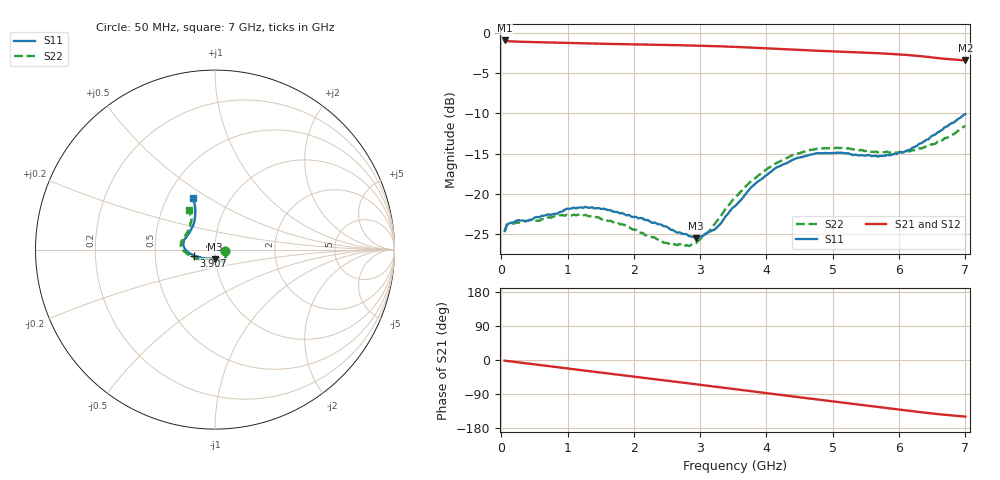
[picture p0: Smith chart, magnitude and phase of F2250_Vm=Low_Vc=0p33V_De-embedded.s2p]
! Integrated Device Technology
! Corporate Headquarters
! 6024 Silver Creek Valley Road
! San Jose, CA 95138  USA
! Phone:  1-408-284-8200
! Toll Free:  1-800-223-1366
! Webpage:  http://www.idt.com/
! Timing and RF Division
! 515 Groton Road, Suite 102
! Westford, MA 01886-6024
! Device:  F2250
! Description: Voltage Variable RF Attenuator
! Frequency:  50.0 -  6000.00 MHz
! Package:  3x3 mm Thin QFN Plastic Package: 16 pin
! Ports:  2 RF, 3 DC
!  Pin  1  = GND
!  Pin  2  = NC
!  Pin  3  = RF1  = Port 1
!  Pin  4  = NC
!  Pin  5  = GND
!  Pin  6  = GND
!  Pin  7  = GND
!  Pin  8  = GND
!  Pin  9  = NC
!  Pin 10  = RF2  = Port 2
!  Pin 11  = NC
!  Pin 12  = GND
!  Pin 13  = GND
!  Pin 14  = VCNTRL
!  Pin 15  = VDD
!  Pin 16  = VMODE
! Vcntrl:  0.330 Volts
! Vmode:  +0.000 Volts
! Vdd:  +3.30  Volts
! Current:  1.119 mA
! Data:  The device was measured on a the F2250 evaluation board which has
!  individual transmission lines to the RF pins.  Data was collected
!  using a calibrated network analyzer.  The evaluation board was
!  de-embedded using a TRL calibration technique.
!  The reference plane is the edge of the package pin.
! Misc:  SN 10
!  Action Tracker AT0258
! Date Measured:  2014-11-26
! Date:  2015-10-15  MJV
! Note:
!  Integrated Device Technology supplies this data as a sample of measured
!  data at the package pin for this product.  Your particular data for this
!  product may vary.
!  Data was taken at 25 degrees C.
!  Integrated Device Technology reserves the right to change this data at anytime.
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# GHz S dB R 50
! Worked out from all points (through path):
!   201 points, 50 MHz to 7 GHz, reference 50 ohm
!   highest |S21| = -0.96 dB at 50 MHz (marker M1); lowest = -3.4 dB at 7 GHz (marker M2)
!   group delay of S21, straight-line fit = 60 ps
!   lowest |S11| = -25.5 dB at 2.934 GHz (marker M3), VSWR 1.11, Z = 49.8 - j5.29 ohm
!   |S11| at or under -10 dB: start of sweep to end of sweep
!   |S22| runs from -26.5 to -11.5 dB; largest |S21 - S12| = 0.00032
!   S11 on the Smith chart (normalised r, x): 50 MHz: 1.12, -0.02; 3.907 GHz: 0.79, -0.05; 7 GHz: 0.67, +0.43
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0.05  -24.58 -9.2  -0.96 -1.8  -0.96 -1.8  -24.72 -9.7
0.08475  -23.77 -9.1  -1.03 -2.5  -1.03 -2.5  -23.84 -9.0
0.15425  -23.54 -11.3  -1.08 -4.0  -1.08 -4.0  -23.61 -10.8
0.57125  -22.88 -28.9  -1.18 -13.1  -1.18 -13.1  -23.34 -29.8
0.884  -22.23 -44.3  -1.24 -19.9  -1.24 -19.9  -22.63 -46.0
1.2315  -21.70 -54.4  -1.32 -27.4  -1.32 -27.4  -22.64 -58.8
1.75275  -22.24 -61.1  -1.41 -38.4  -1.41 -38.4  -23.47 -66.1
2.37825  -23.76 -62.1  -1.50 -51.8  -1.50 -51.8  -25.70 -68.5
2.552  -24.41 -66.1  -1.53 -55.6  -1.53 -55.6  -26.33 -74.2
2.83  -25.22 -80.7  -1.58 -61.7  -1.58 -61.7  -26.45 -92.9
2.93425  -25.51 -89.4  -1.60 -64.0  -1.60 -64.0  -26.11 -101.4
3.21225  -24.44 -118.6  -1.66 -70.2  -1.66 -70.2  -23.77 -126.7
3.525  -21.50 -145.8  -1.76 -77.1  -1.76 -77.1  -20.48 -145.7
3.76825  -19.17 -159.5  -1.85 -82.5  -1.85 -82.5  -18.39 -156.2
3.90725  -18.26 -164.0  -1.90 -85.5  -1.90 -85.5  -17.52 -162.3
4.1505  -16.70 -172.4  -2.00 -90.8  -2.00 -90.8  -16.16 -171.0
4.7065  -15.05 173.2  -2.21 -102.9  -2.21 -102.9  -14.51 175.9
5.15825  -14.91 162.5  -2.37 -112.6  -2.37 -112.6  -14.27 166.7
5.85325  -15.20 139.2  -2.62 -127.5  -2.62 -127.5  -14.88 151.6
6.166  -14.52 128.2  -2.79 -134.3  -2.79 -134.4  -14.70 142.7
6.444  -13.20 119.8  -3.00 -140.1  -3.00 -140.1  -14.09 133.3
7  -10.09 113.4  -3.44 -149.4  -3.44 -149.4  -11.55 123.8
